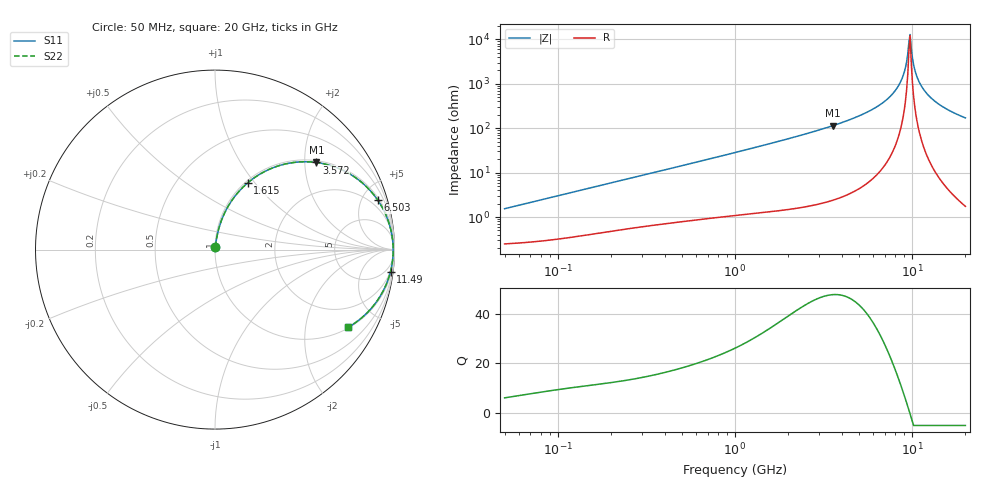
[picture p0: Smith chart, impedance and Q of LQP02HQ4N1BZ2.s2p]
!Murata Part Number: LQP02HQ4N1BZ2
!These Parameters are Measured in Series Mode Connection
!  o--[Z]--o
!Port1  Port2
!  o-------o
!Freq. Start=50[MHz] Stop=20[GHz], 401[Steps]
# Hz S RI R 50
!Freq.(Hz) S11(Real) S11(Imag) S21(Real) S21(Imag) S12(Real) S12(Imag) S22(Real) S22(Imag)
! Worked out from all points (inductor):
!   401 points, 50 MHz to 20 GHz, reference 50 ohm
!   read as one part in series: L = 4.83 nH near 51.52 MHz
!   highest Q = 47.7 at 3.572 GHz (marker M1), where L = 5.09 nH
!   self-resonance near 9.6 GHz
!   S11 on the Smith chart (normalised r, x): 50 MHz: 1.00, +0.03; 1.615 GHz: 1.03, +0.92; 3.572 GHz: 1.05, +2.28; 6.503 GHz: 1.20, +6.51; 11.49 GHz: 2, -16; 20 GHz: 1.03, -3.41
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5e7  0.00271 0.0152  0.9973 -0.0152  0.9973 -0.0152  0.00271 0.0152
1.364002e8  0.00542 0.0404  0.9946 -0.0404  0.9946 -0.0404  0.00542 0.0404
3.721004e8  0.0178 0.1044  0.9822 -0.1044  0.9822 -0.1044  0.0178 0.1044
1e9  0.0826 0.2568  0.9174 -0.2568  0.9174 -0.2568  0.0826 0.2568
1.614971e9  0.1828 0.3723  0.8172 -0.3723  0.8172 -0.3723  0.1828 0.3723
2.728004e9  0.4042 0.4798  0.5958 -0.4798  0.5958 -0.4798  0.4042 0.4798
3.572216e9  0.5649 0.4854  0.4351 -0.4854  0.4351 -0.4854  0.5649 0.4854
5.041459e9  0.779 0.4035  0.221 -0.4035  0.221 -0.4035  0.779 0.4035
6.503449e9  0.9068 0.2757  0.0932 -0.2757  0.0932 -0.2757  0.9068 0.2757
7.442007e9  0.9537 0.1898  0.0463 -0.1898  0.0463 -0.1898  0.9537 0.1898
8.141811e9  0.9752 0.1278  0.0248 -0.1278  0.0248 -0.1278  0.9752 0.1278
8.774992e9  0.9867 0.0742  0.0133 -0.0742  0.0133 -0.0742  0.9867 0.0742
9.178299e9  0.9908 0.0414  0.00924 -0.0414  0.00924 -0.0414  0.9908 0.0414
9.457416e9  0.9922 0.0195  0.00778 -0.0195  0.00778 -0.0195  0.9922 0.0195
9.745021e9  0.9927 -0.0025  0.0073 0.0025  0.0073 0.0025  0.9927 -0.0025
9.892087e9  0.9926 -0.0135  0.00742 0.0135  0.00742 0.0135  0.9926 -0.0135
1.019291e10  0.9916 -0.0355  0.00841 0.0355  0.00841 0.0355  0.9916 -0.0355
1.050288e10  0.9896 -0.0574  0.0104 0.0574  0.0104 0.0574  0.9896 -0.0574
1.149051e10  0.9779 -0.1224  0.0221 0.1224  0.0221 0.1224  0.9779 -0.1224
1.257102e10  0.9576 -0.1851  0.0424 0.1851  0.0424 0.1851  0.9576 -0.1851
1.417136e10  0.9182 -0.2632  0.0818 0.2632  0.0818 0.2632  0.9182 -0.2632
2e10  0.7417 -0.4326  0.2583 0.4326  0.2583 0.4326  0.7417 -0.4326
